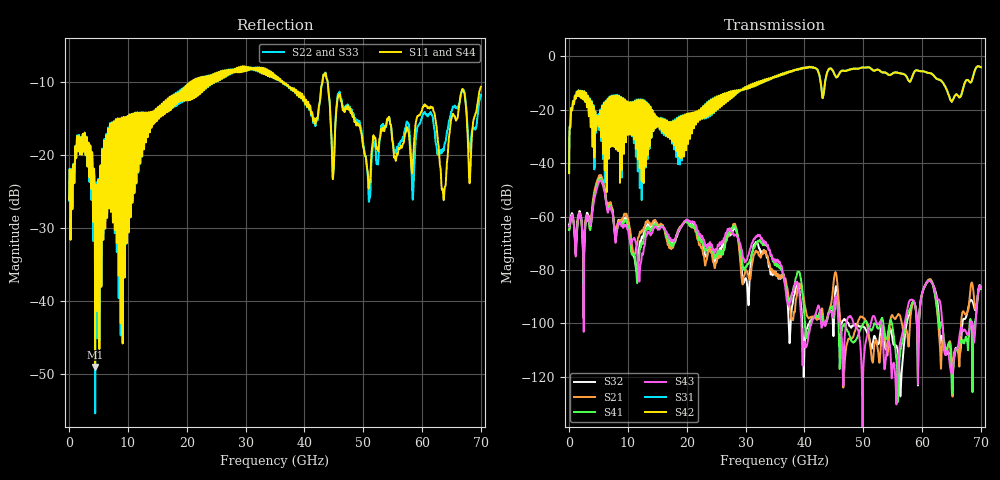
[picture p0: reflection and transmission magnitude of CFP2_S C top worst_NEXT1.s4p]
! AWR Design Environment (8415) Tue Jan 08 13:15:12 2019
! Document = 'CFP2 Channel_S'
! nPorts: 4, nXvals: 7001
# HZ S DB R 50
!Freq DBS11 AngS11 DBS12 AngS12 DBS13 AngS13 DBS14 AngS14
!	DBS21 AngS21 DBS22 AngS22 DBS23 AngS23 DBS24 AngS24
!	DBS31 AngS31 DBS32 AngS32 DBS33 AngS33 DBS34 AngS34
!	DBS41 AngS41 DBS42 AngS42 DBS43 AngS43 DBS44 AngS44
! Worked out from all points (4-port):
!   7000 points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, 10 MHz to 70 GHz, reference 50 ohm
!   strongest paths, dB at 10 MHz, 17.51 GHz, 35.01 GHz, 52.51 GHz, 70 GHz:
!     S42: -43.7, -31.9, -7.5, -5.0, -4.0
!     S31: -43.4, -32.7, -7.5, -5.0, -4.0
!     S43: -63.6, -68.8, -76.7, -100.4, -86.7
!     S41: -65.0, -70.3, -78.1, -101.9, -87.2
!     S21: -64.9, -71.0, -81.4, -110.0, -86.9
!     S32: -63.1, -69.6, -81.2, -107.8, -86.5
!   lowest |S11| = -49.0 dB at 4.43 GHz (marker M1), VSWR 1.01, Z = 49.9 + j0.337 ohm
!   |S11| at or under -10 dB: start of sweep to 20.77 GHz; 36.28 GHz to 43.07 GHz (6.792 GHz wide, 17.1 % of centre); 43.96 GHz to end of sweep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
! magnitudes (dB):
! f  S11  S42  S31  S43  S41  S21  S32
! 10 MHz  -26.1  -43.7  -43.4  -63.6  -65.0  -64.9  -63.1
! 1.32 GHz  -18.0  -13.3  -13.2  -67.1  -66.5  -64.9  -65.7
! 4.43 GHz  -49.0  -21.0  -20.4  -52.2  -51.1  -49.2  -50.3
! 11.55 GHz  -14.8  -16.7  -16.4  -73.0  -84.7  -70.4  -79.7
! 19.94 GHz  -12.3  -27.1  -26.4  -61.1  -61.7  -61.8  -61.3
! 29.7 GHz  -8.6  -12.5  -12.4  -75.7  -79.1  -82.4  -84.7
! 70 GHz  -10.7  -4.0  -4.0  -86.7  -87.2  -86.9  -86.5
